// ------------------------------------------------------------------
// File           : C:\Users\acer\Documents\hla.awl
//
// Source File    : C:\Users\acer\Documents\hla.var
// Generation Date: 12/4/2018  Time: 11:40:03 AM
// ------------------------------------------------------------------

DATA_BLOCK DB  122
VERSION : 0.0


STRUCT

 V3_M_r0067_67:
   STRUCT
   SYNTAX_ID : BYTE := B#16#82;
   bereich_u_einheit : BYTE := B#16#A3;
   spalte : WORD := W#16#43;
   zeile : WORD := W#16#1;
   bausteintyp : BYTE := B#16#1A;
   ZEILENANZAHL : BYTE := B#16#1;
   typ : BYTE := B#16#8;
   laenge : BYTE := B#16#4;
   END_STRUCT ;

 V3_M_r0068_68:
   STRUCT
   SYNTAX_ID : BYTE := B#16#82;
   bereich_u_einheit : BYTE := B#16#A3;
   spalte : WORD := W#16#44;
   zeile : WORD := W#16#1;
   bausteintyp : BYTE := B#16#1A;
   ZEILENANZAHL : BYTE := B#16#1;
   typ : BYTE := B#16#8;
   laenge : BYTE := B#16#4;
   END_STRUCT ;

 END_STRUCT ;

BEGIN
END_DATA_BLOCK
